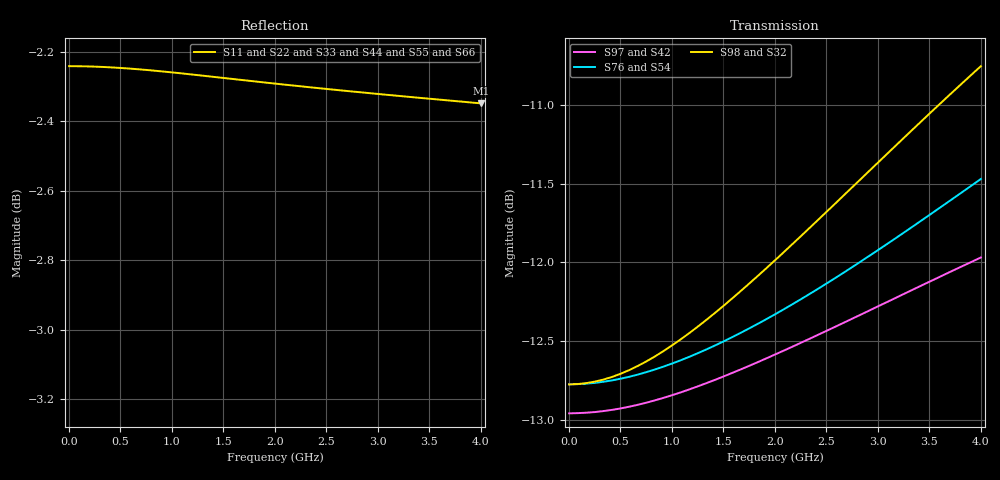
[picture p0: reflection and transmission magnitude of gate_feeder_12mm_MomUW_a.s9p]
! Created Thu Sep 17 15:56:48 2015
# ghz S ma R 50
! 9 Port Network Data from data block
! freq  magS11  angS11  magS12  angS12  magS13  angS13  magS14  angS14
!  magS15  angS15  magS16  angS16  magS17  angS17  magS18  angS18
!  magS19  angS19
!  magS21  angS21  magS22  angS22  magS23  angS23
!  magS24  angS24  magS25  angS25  magS26  angS26  magS27  angS27
!  magS28  angS28  magS29  angS29
!  magS31  angS31  magS32  angS32
!  magS33  angS33  magS34  angS34  magS35  angS35  magS36  angS36
!  magS37  angS37  magS38  angS38  magS39  angS39
!  magS41  angS41
!  magS42  angS42  magS43  angS43  magS44  angS44  magS45  angS45
!  magS46  angS46  magS47  angS47  magS48  angS48  magS49  angS49
!  magS51  angS51  magS52  angS52  magS53  angS53  magS54  angS54
!  magS55  angS55  magS56  angS56  magS57  angS57  magS58  angS58
!  magS59  angS59
!  magS61  angS61  magS62  angS62  magS63  angS63
!  magS64  angS64  magS65  angS65  magS66  angS66  magS67  angS67
!  magS68  angS68  magS69  angS69
!  magS71  angS71  magS72  angS72
!  magS73  angS73  magS74  angS74  magS75  angS75  magS76  angS76
!  magS77  angS77  magS78  angS78  magS79  angS79
!  magS81  angS81
!  magS82  angS82  magS83  angS83  magS84  angS84  magS85  angS85
!  magS86  angS86  magS87  angS87  magS88  angS88  magS89  angS89
!  magS91  angS91  magS92  angS92  magS93  angS93  magS94  angS94
!  magS95  angS95  magS96  angS96  magS97  angS97  magS98  angS98
!  magS99  angS99
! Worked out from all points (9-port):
!   50 points, 1 MHz to 4 GHz, reference 50 ohm
!   strongest paths, dB at 1 MHz, 917.4 MHz, 2.001 GHz, 3 GHz, 4 GHz:
!     S98: -12.8, -12.6, -12.0, -11.4, -10.7
!     S32: -12.8, -12.6, -12.0, -11.4, -10.8
!     S76: -12.8, -12.7, -12.3, -11.9, -11.5
!     S54: -12.8, -12.7, -12.3, -11.9, -11.5
!     S97: -13.0, -12.9, -12.6, -12.3, -12.0
!     S42: -13.0, -12.9, -12.6, -12.3, -12.0
!   lowest |S11| = -2.3 dB at 4 GHz (marker M1), VSWR 7.44, Z = 6.73 + j1.94 ohm
!   |S11| at or under -10 dB: nowhere
